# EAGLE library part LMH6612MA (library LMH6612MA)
Output Amplifiers Source: Datasheet
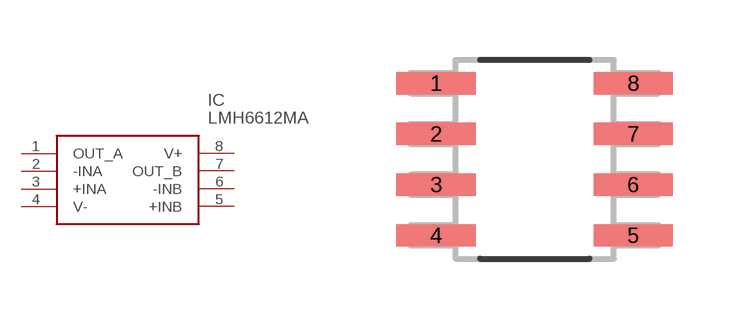
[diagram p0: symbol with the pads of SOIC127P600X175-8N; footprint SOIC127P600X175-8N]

Designator prefix IC

## LMH6612MA (Description: Output Amplifiers; Height: mm; Manufacturer_Name: Texas Instruments; Manufacturer_Part_Number: LMH6612MA)  [SOIC127P600X175-8N]
1  OUT_A
2  -INA
3  +INA
4  V-
5  +INB
6  -INB
7  OUT_B
8  V+

## Footprint SOIC127P600X175-8N (pad centres in mm)
SOIC127P600X175-8N
smd 1.981 x 0.559: 1 -2.464,1.905; 2 -2.464,0.635; 3 -2.464,-0.635; 4 -2.464,-1.905; 5 2.464,-1.905; 6 2.464,-0.635; 7 2.464,0.635; 8 2.464,1.905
